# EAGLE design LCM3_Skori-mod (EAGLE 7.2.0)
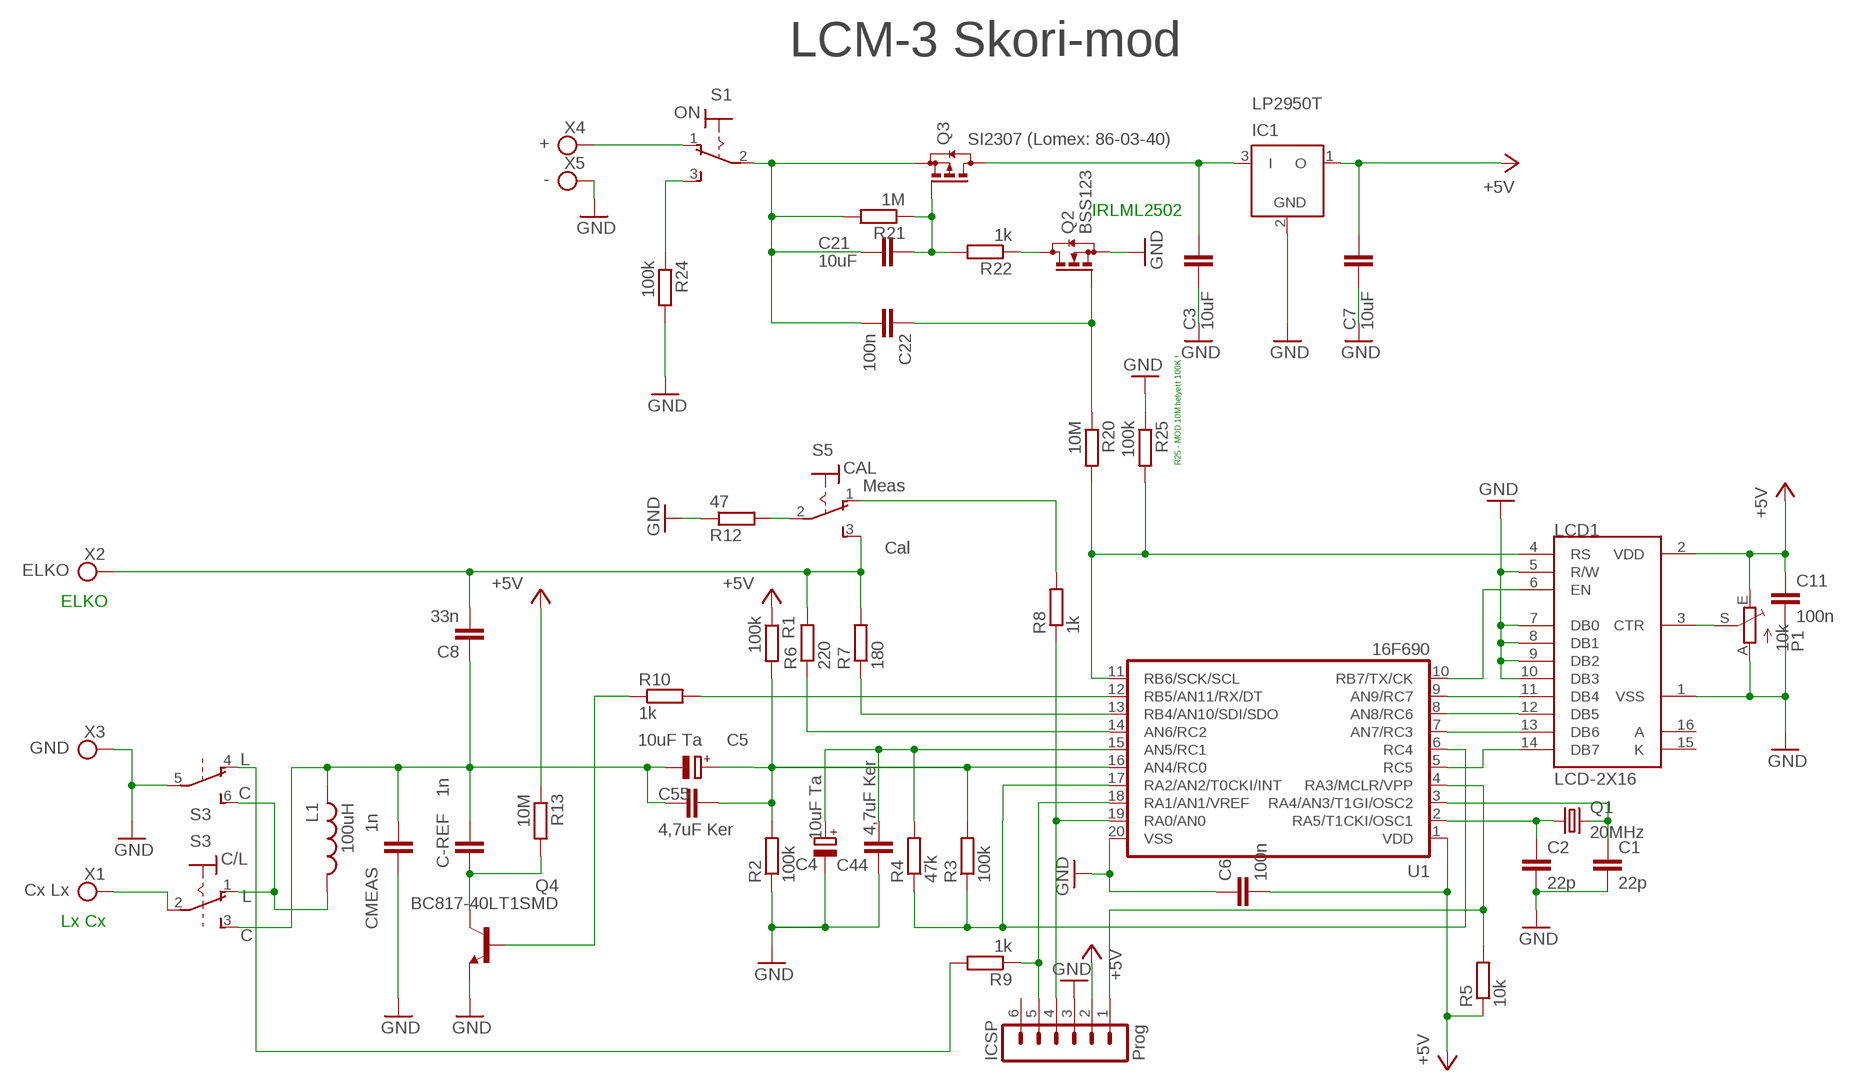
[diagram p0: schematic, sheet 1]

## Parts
C1  22p  C-EUC1206K  [C1206K]
C2  22p  C-EUC1206K  [C1206K]
C3  10uF  C-EUC1206K  [C1206K]
C4  10uF Ta  CPOL-EU085CS-1AR  [085CS_1AR]
C5  10uF Ta  CPOL-EU085CS-1AR  [085CS_1AR]
C6  100n  C-EUC1206K  [C1206K]
C7  10uF  C-EUC1206K  [C1206K]
C8  33n  C-EU102-064X133  [C102-064X133]
C11  100n  C-EUC1206K  [C1206K]
C21  10uF  C-EUC1206K  [C1206K]
C22  100n  C-EUC1206K  [C1206K]
C44  4,7uF Ker  C-EUC1206K  [C1206K]
C55  4,7uF Ker  C-EUC1206K  [C1206K]
C-REF  1n  C-EU102-064X133  [C102-064X133]
CMEAS  1n  C-EU102-064X133  [C102-064X133]
IC1  LP2950T  [TO92-T]
ICSP  Prog  MA06-1  [MA06-1]
L1  100uH  L-USTJ3-U2  [TJ3-U2]
LCD1  LCD-2X16  LCD-2X16,  [MTB-086]
P1  10k  TRIM_EU-CA9V  [CA9V]
Q1  20MHz  CRYSTALHC49U70  [HC49U70]
Q2  BSS123  [SOT23]
Q3  SI2307 (Lomex: 86-03-40)  BSS84  [SOT23]
Q4  BC817-40LT1SMD  [SOT23-BEC]
R1  100k  R-EU_R1206  [R1206]
R2  100k  R-EU_R1206  [R1206]
R3  100k  R-EU_R1206  [R1206]
R4  47k  R-EU_R1206  [R1206]
R5  10k  R-EU_R1206  [R1206]
R6  220  R-EU_R1206  [R1206]
R7  180  R-EU_R1206  [R1206]
R8  1k  R-EU_R1206  [R1206]
R9  1k  R-EU_R1206  [R1206]
R10  1k  R-EU_R1206  [R1206]
R12  47  R-EU_R2512  [R2512]
R13  10M  R-EU_R1206  [R1206]
R20  10M  R-EU_R1206  [R1206]
R21  1M  R-EU_R1206  [R1206]
R22  1k  R-EU_R1206  [R1206]
R24  100k  R-EU_R1206  [R1206]
R25  100k  R-EU_R1206  [R1206]
S1  ON  M9040P  [M9040P]
S3  C/L  M9040P2,  [M9040P2B]
S5  CAL  M9040P  [M9040P]
U1  16F690  PIC16F6XX  [DIL20]
X1  Cx Lx  PIN1,3-121  [PIN-4]
X2  ELKO  PIN1,3-121  [PIN-4]
X3  GND  PIN1,3-121  [PIN-4]
X4  +  PIN1,3-121  [PIN-4]
X5  -  PIN1,3-121  [PIN-4]

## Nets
+5V: C6.2 C7.1 C11.1 IC1.1(O) ICSP.2 LCD1.2(VDD) P1.E R1.1 R5.1 R13.1 U1.1(VDD)
GND: C1.2 C2.2 C3.2 C4.- C6.1 C7.2 C11.2 C44.1 CMEAS.1 IC1.2(GND) ICSP.3 LCD1.1(VSS) LCD1.5(R/W) LCD1.7(DB0) LCD1.8(DB1) LCD1.9(DB2) LCD1.10(DB3) P1.A Q2.2(S) Q4.E R2.1 R12.1 R24.2 R25.1 S3.5(2:P) U1.20(VSS) X3.1(KL) X5.1(KL)
N$1: LCD1.14(DB7) U1.5(RC5)
N$2: LCD1.13(DB6) U1.7(AN7/RC3)
N$3: LCD1.12(DB5) U1.8(AN8/RC6)
N$4: LCD1.11(DB4) U1.9(AN9/RC7)
N$5: LCD1.3(CTR) P1.S
N$6: LCD1.4(RS) R20.2 R25.2 U1.11(RB6/SCK/SCL)
N$7: LCD1.6(EN) U1.10(RB7/TX/CK)
N$8: C1.1 Q1.2 U1.3(RA4/AN3/T1GI/OSC2)
N$9: C2.1 Q1.1 U1.2(RA5/T1CKI/OSC1)
N$10: R24.1 S1.3(S)
N$11: R3.1 R4.1 U1.6(RC4) U1.17(RA2/AN2/T0CKI/INT)
N$12: C4.+ C44.2 R4.2 U1.15(AN5/RC1)
N$13: C5.- C8.1 C55.2 C-REF.2 CMEAS.2 L1.2 S3.3(1:S)
N$14: C8.2 R6.2 R7.2 S5.3(S) X2.1(KL)
N$15: R10.2 U1.12(RB5/AN11/RX/DT)
N$16: R6.1 U1.14(AN6/RC2)
N$17: C-REF.1 Q4.C R13.2
N$18: R7.1 U1.13(RB4/AN10/SDI/SDO)
N$19: ICSP.4 R8.1 U1.19(RA0/AN0)
N$20: R8.2 S5.1(O)
N$21: R12.2 S5.2(P)
N$22: ICSP.5 R9.1 U1.18(RA1/AN1/VREF)
N$23: R9.2 S3.4(2:O)
N$24: L1.1 S3.1(1:O) S3.6(2:S)
N$25: C5.+ C55.1 R1.2 R2.2 R3.2 U1.16(AN4/RC0)
N$26: S3.2(1:P) X1.1(KL)
N$27: ICSP.1 R5.2 U1.4(RA3/MCLR/VPP)
N$28: S1.1(O) X4.1(KL)
N$29: C3.1 IC1.3(I) Q3.3(D)
N$30: Q2.3(D) R22.1
N$31: C21.1 Q3.1(G) R21.1 R22.2
N$32: C21.2 C22.2 Q3.2(S) R21.2 S1.2(P)
N$34: C22.1 Q2.1(G) R20.1
N$37: Q4.B R10.1
Unconnected: ICSP.6

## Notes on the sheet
- LCM-3 Skori-mod
- IRLML2502
- R25 - MOD 10M helyett 100K !
- Meas
- Cal
- ELKO
- L
- C
- L
- Lx Cx
- C

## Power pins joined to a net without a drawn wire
A: LCD1.16(A)
K: LCD1.15(K)

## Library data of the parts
C1-C3 C6-C8 C11 C21 C22 C44 C55 C-REF CMEAS = rcl:C-EU: CAPACITOR, European symbol
C4 C5 = rcl:CPOL-EU: POLARIZED CAPACITOR, European symbol
IC1 = linear:LP2950: 100 mA, Low Power Low Dropout Voltage Regulator Source: http://www.onsemi.com/pub/Collateral/LP2950-D.PDF
ICSP = con-lstb:MA06-1: PIN HEADER
L1 = rcl:L-US: INDUCTOR, American symbol
LCD1 = 01_LCM3:LCD-2X16: LCD kijelzö
P1 = pot:TRIM_EU-: POTENTIOMETER
Q1 = crystal:CRYSTAL: CRYSTAL
Q2 = transistor-small-signal:BSS123: N-CHANNEL MOS FET
Q3 = transistor-small-signal:BSS84: P-CHANNEL MOS FET
Q4 = transistor-npn:BC817*: NPN Transistor
R1-R10 R12 R13 R20-R22 R24 R25 = rcl:R-EU_: RESISTOR, European symbol
S1 S5 = switch:M9040P: TOGGLE SWITCH Marquardt
S3 = 01_LCM3:M9040P2: TOGGLE SWITCH Marquardt
U1 = pic16f690:PIC16F6XX
X1-X5 = 01skori-hp:PIN: CONNECTOR

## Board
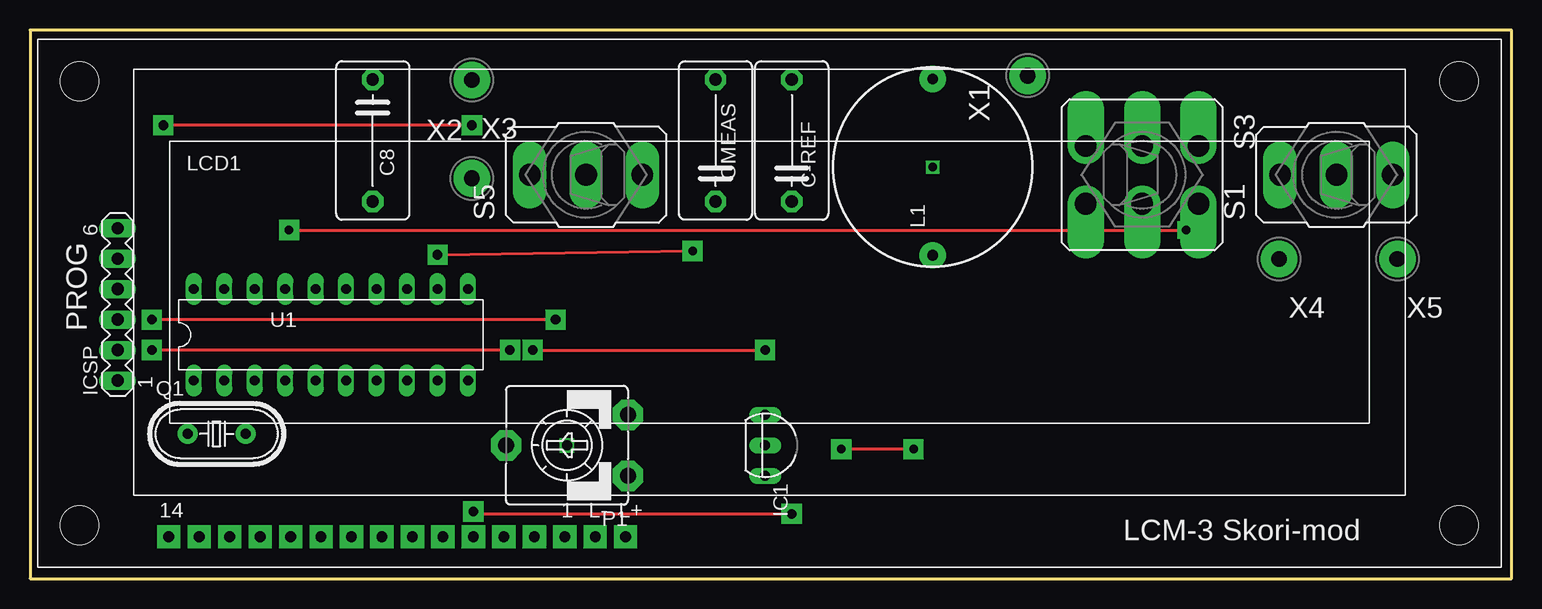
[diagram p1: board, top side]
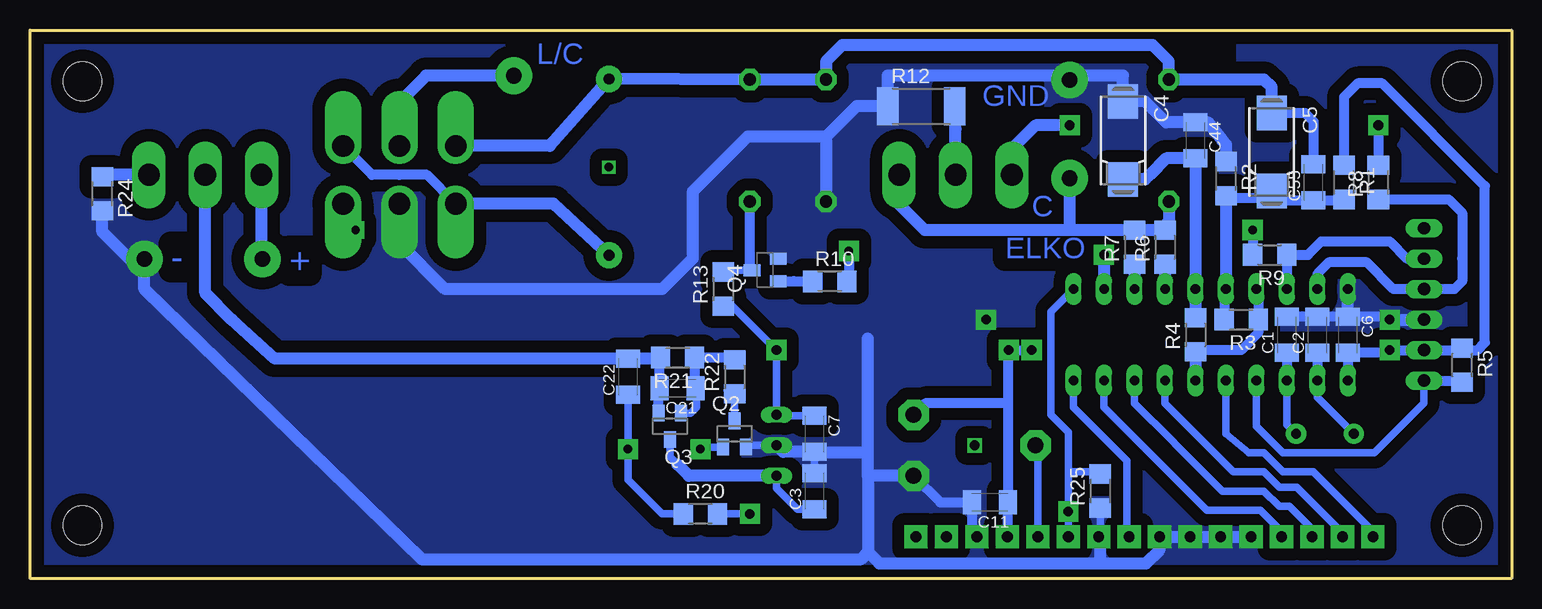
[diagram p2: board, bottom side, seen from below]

Size 123.51 x 45.72 mm. Coordinates in mm from the lower left corner, seen from the top.
Outline: 0,0 123.51,0 123.51,45.72 0,45.72 0,0
Copper layers (1*16): Top 0.035mm / dielectric 1.5mm / Bottom 0.035mm
Design rules "default": minimum track width 10mil, minimum drill 24mil, track to track 8mil, track to pad 8mil, pad to pad 8mil, via to via 8mil, smd to smd 8mil, copper to edge 40mil, drill to drill 8mil, minimum pad ring 10mil, minimum via ring 8mil, stop-mask expansion 4mil, vias tented up to drill 0mil, thermal gap 10mil

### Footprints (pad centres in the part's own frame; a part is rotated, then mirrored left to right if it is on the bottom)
C1206K = smd 1.5 x 2: 1 -1.5,0; 2 1.5,0
085CS_1AR = smd 2.9 x 2.5: + 3.25,0; - -3.25,0
C102-064X133 = drill 1.016 pad 1.778 octagon: 1 -5.08,0; 2 5.08,0
TO92-T = drill 0.813 long: 1 -2.54,0; 2 0,0; 3 2.54,0
MA06-1 = drill 1.016 long: 1 -6.35,0; 2 -3.81,0; 3 -1.27,0; 4 1.27,0; 5 3.81,0; 6 6.35,0
TJ3-U2 = drill 0.9 pad 2.184: 1 -7.35,0; 2 7.35,0
MTB-086 = drill 0.9 pad 1.93 square: 1 43.942,2.54; 2 41.402,2.54; 3 38.862,2.54; 4 36.322,2.54; 5 33.782,2.54; 6 31.242,2.54; 7 28.702,2.54; 8 26.162,2.54; 9 23.622,2.54; 10 21.082,2.54; 11 18.542,2.54; 12 16.002,2.54; 13 13.462,2.54; 14 10.922,2.54; 15 46.482,2.54; 16 49.022,2.54 | hole 3.2: 3.5,3.5; 3.5,40.5; 118.5,40.5; 118.5,3.5
CA9V = drill 1.321 pad 2.54 octagon: A -2.54,-5.08; E 2.54,-5.08; S 0,5.08
HC49U70 = drill 0.813 pad 1.676: 1 -2.413,0; 2 2.413,0
SOT23 = smd 1 x 1.4: 1 -0.95,-1.1; 2 0.95,-1.1; 3 0,1.1
SOT23-BEC = smd 1 x 1.4: B -0.95,-1.1; C 0,1.1; E 0.95,-1.1
R1206 = smd 1.6 x 1.803: 1 -1.422,0; 2 1.422,0
R2512 = smd 1.8 x 3.2: 1 -2.8,0; 2 2.8,0
M9040P = drill 1.803 pad 2.794 long: 1 0,4.699; 2 0,0; 3 0,-4.699
M9040P2B = drill 1.803 pad 3.048 offset: 1 -2.413,4.699; 2 -2.413,0; 3 -2.413,-4.699; 4 2.413,4.699; 5 2.413,0; 6 2.413,-4.699
DIL20 = drill 0.813 long: 1 -11.43,-3.81; 2 -8.89,-3.81; 3 -6.35,-3.81; 4 -3.81,-3.81; 5 -1.27,-3.81; 6 1.27,-3.81; 7 3.81,-3.81; 8 6.35,-3.81; 9 8.89,-3.81; 10 11.43,-3.81; 11 11.43,3.81; 12 8.89,3.81; 13 6.35,3.81; 14 3.81,3.81; 15 1.27,3.81; 16 -1.27,3.81; 17 -3.81,3.81; 18 -6.35,3.81; 19 -8.89,3.81; 20 -11.43,3.81
PIN-4 = drill 1.3 pad 3.048: 1 0,0.025

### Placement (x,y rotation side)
C1  18.73,20.32 90 bottom
C2  16.19,20.32 90 bottom
C3  58.1,7.3 90 bottom
C4  32.39,36.51 270 bottom
C5  20,35.56 270 bottom
C6  13.65,20.32 270 bottom
C7  58.1,12.06 270 bottom
C8  28.58,36.51 270 top
C11  43.5,6.35 180 bottom
C21  69.53,15.88 180 bottom
C22  73.66,16.83 90 bottom
C44  26.35,36.51 270 bottom
C55  16.51,33.02 90 bottom
C-REF  63.5,36.51 90 top
CMEAS  57.15,36.51 90 top
IC1  61.28,11.11 270 top
ICSP  7.3,22.86 90 top
L1  75.25,34.29 90 top
LCD1  0.64,0.95 0 top
P1  44.77,11.11 90 top
Q1  15.56,12.06 0 top
Q2  64.77,12.06 0 bottom
Q3  70.17,12.7 180 bottom
Q4  62.23,25.72 90 bottom
R1  13.97,33.02 270 bottom
R2  23.81,33.34 270 bottom
R3  22.54,21.59 180 bottom
R4  26.35,20.32 90 bottom
R5  4.13,17.78 270 bottom
R6  28.89,27.62 90 bottom
R7  31.43,27.62 90 bottom
R8  11.11,33.02 90 bottom
R9  20.16,26.99 180 bottom
R10  56.83,24.77 0 bottom
R12  49.21,39.37 0 bottom
R13  65.72,24.13 90 bottom
R20  67.63,5.4 0 bottom
R21  69.53,18.41 180 bottom
R22  64.77,16.83 90 bottom
R24  117.47,32.07 270 bottom
R25  34.29,7.3 90 bottom
S1  108.9,33.65 90 top
S3  92.71,33.65 270 top
S5  46.36,33.65 90 top
U1  25.08,20.32 0 top
X1  83.19,41.91 90 top
X2  36.83,33.34 0 top
X3  36.83,41.59 180 top
X4  104.14,26.67 180 top
X5  113.98,26.67 180 top

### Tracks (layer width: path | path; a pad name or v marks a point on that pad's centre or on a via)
+5V  (via drill 0.8 pad 1.68)
  Top 0.254: v40,19.05 v10.16,19.05 | v41.91,19.05 v61.28,19.05
  Bottom 0.61: C11.1 42.04,6.39 42.04,6.98 | C7.1 61.19,13.56 IC1.1 v61.28,19.05 64.94,22.71 R13.1
  Bottom 0.813: R1.1 13.97,40.13 12.83,41.27 10.8,41.27 2.22,32.7 2.22,19.68 2.86,19.05 3.66,19.05 R5.1 3.81,19.05 ICSP.2 v10.16,19.05 10.16,18.82 C6.2 U1.1 | 42,14.6 42,19.05 v41.91,19.05 v40,19.05 | 42,14.6 C11.1 | P1.E 48.9,14.6 42,14.6 | 42.04,6.98 LCD1.2
GND  (via drill 0.8 pad 1.68)
  Top 0.254: v43.81,21.59 v10.16,21.59
  Bottom 0.61: C11.2 44.58,5.93 | C7.2 58.1,10.48 C3.2 | R25.1 34.29,3.49 LCD1.5 | 73.34,1.59 73.49,1.59 | Q2.2 63.67,11.11 IC1.2
  Bottom 0.813: C4.- 32.46,39.76 | C1.2 C2.2 C6.1 10.16,21.82 v10.16,21.59 | 34.29,3.37 LCD1.5 | P1.A 47.62,6.35 C11.2 45,3.49 LCD1.1
  Bottom 1.016: LCD1.10 LCD1.9 LCD1.8 LCD1.7 29.34,2.41 30.48,1.27 34.29,1.27 | C6.1 U1.20 | v10.16,21.59 ICSP.3 | 23.81,34.61 R2.1 23.81,36.2 24.13,36.51 25.31,38.01 C44.1 28.81,38.01 30.56,39.76 C4.- 32.39,41.91 36.17,41.91 | 36.17,41.91 X3.1 | 36.17,41.91 52.01,41.91 R12.1 54.61,39.37 57.15,36.83 | 57.15,36.83 CMEAS.1 | 34.29,1.27 52.7,1.27 53.66,2.22 | 53.66,10.48 53.66,20 | 53.66,8.57 53.66,10.48 | 53.66,8.57 53.66,2.22 | P1.A 53.66,8.57 | 34.29,1.27 34.29,3.37 | 53.66,2.22 54.29,1.59 73.34,1.59 90.81,1.59 113.98,24.13 X5.1 114.01,26.67 115.25,26.67 117.47,28.89 R24.2 | IC1.2 60.73,10.56 C7.2 | 53.66,10.48 58.1,10.48 | S3.5 92.71,27.94 88.9,24.13 70.8,24.13 68.26,26.67 68.26,32.25 63.68,36.83 57.15,36.83
  pour Bottom (isolate 1.016, no thermals): 0.95,44.45 122.24,44.45 122.24,0.63 0.95,0.63
N$1
  Bottom 0.61: LCD1.14 11.75,3.68 11.75,4.13 16.51,8.89 19.05,8.89 20.64,10.48 21.91,10.48 23.81,12.06 23.81,13.65 U1.5
N$2
  Bottom 0.61: LCD1.13 14.29,3.68 14.29,4 17.91,7.62 19.05,7.62 19.37,7.62 20.64,8.89 23.18,8.89 26.35,12.06 27.31,13.02 28.89,14.6 28.89,15.24 U1.7
N$3
  Bottom 0.61: LCD1.12 16.83,3.68 16.83,4.32 18.54,6.03 18.73,6.03 19.37,6.03 20.64,7.3 21.91,7.3 24.13,7.3 27.94,11.11 28.26,11.43 31.43,14.6 U1.8
N$4
  Bottom 0.61: U1.9 33.97,14.29 29.53,9.84 25.4,5.72 20.95,5.72 19.69,4.45 19.18,3.94 LCD1.11
N$5
  Bottom 0.61: P1.S 39.5,10.92 LCD1.3
N$6  (via drill 0.8 pad 1.68)
  Top 0.254: 37.15,5.4 v63.5,5.4
  Top 0.61: v36.96,5.59 37.15,5.4
  Bottom 0.61: U1.11 38.42,22.23 38.42,21.59 38.42,13.65 36.96,12.19 36.96,8.89 | 36.96,8.89 v36.96,5.59 LCD1.4 | R25.2 34.29,8.89 36.96,8.89 | v63.5,5.4 R20.2
N$7
  Bottom 0.61: LCD1.6 32.07,3.68 32.07,9.84 36.51,14.29 U1.10
N$8
  Bottom 0.61: Q1.2 18.73,12.83 U1.3
  Bottom 0.813: C1.1 U1.3
N$9
  Bottom 0.61: Q1.1 16.19,15.11 U1.2
  Bottom 0.813: C2.1 U1.2
N$10
  Bottom 1.016: R24.1 117.31,33.65 S1.3
N$11
  Bottom 0.813: U1.17 21.12,23.98 R3.1 21.12,20.47 22.54,19.05 23.02,19.05 26.2,19.05 R4.1
  Bottom 1.016: R4.1 26.35,17.78 U1.6
N$12
  Bottom 1.016: R4.2 26.35,22.23 U1.15 C44.2 28.81,35.01 30.16,33.65 30.56,33.26 C4.+
N$13
  Bottom 0.813: 57.15,41.91 CMEAS.2 | C5.- 17.22,38.81 16.51,38.1 C55.2
  Bottom 1.016: CMEAS.2 C-REF.2 L1.2 80.18,36.07 S3.3 | 57.15,41.91 57.15,43.1 55.8,44.45 29.92,44.45 28.58,43.1 C8.1 20.64,41.59 20,40.96 C5.-
N$14
  Bottom 0.813: R6.2 28.89,29.53 28.58,29.85
  Bottom 1.016: R6.2 R7.2 33.17,29.04 36.83,29.04 | C8.2 28.58,29.85 | X2.1 36.83,30.48 36.83,29.04 | S5.3 51.05,31.19 48.91,29.04 36.83,29.04
N$15  (via drill 0.7 pad 1.68, 0.8 pad 1.68)
  Top 0.254: v33.97,26.99 v55.24,27.3
  Bottom 0.813: v55.24,27.3 55.24,24.93 R10.2
  Bottom 1.016: v33.97,26.99 U1.12
N$16
  Bottom 1.016: R6.1 U1.14
N$17
  Bottom 0.61: 63.5,25.72 65.56,25.72 arc-90 R13.2
  Bottom 0.813: Q4.C 63.5,25.72 C-REF.1
N$18
  Bottom 1.016: R7.1 U1.13
N$19
  Bottom 0.813: U1.19 16.19,25.4 15.24,26.35 12.06,26.35 9.84,24.13 ICSP.4 4.76,24.13 4.13,24.77 4.13,26.67 4.13,30.48 5.25,31.6 R8.1
N$20  (via drill 0.8 pad 1.68)
  Top 0.254: v36.83,37.78 v11.11,37.78
  Bottom 0.813: v11.11,37.78 R8.2
  Bottom 1.016: v36.83,37.78 39.69,37.78 41.59,35.88 S5.1
N$21
  Bottom 1.016: R12.2 46.36,37.46 S5.2
N$22
  Bottom 0.813: U1.18 R9.1 16.99,26.99 15.88,28.1 14.76,28.1 10.16,28.1 8.73,26.67 ICSP.5
N$23  (via drill 0.7 pad 1.42, 0.7 pad 1.68)
  Top 0.254: v21.59,29.05 v96.36,29.05
  Bottom 0.813: R9.2 21.59,28.58 v21.59,29.05
  Bottom 1.016: S3.4 96.36,29.02 v96.36,29.05
N$24
  Bottom 0.813: S3.1 95,33.65 92.71,33.65 90.42,33.65 S3.6
  Bottom 1.016: S3.6 87.76,31.24 79.87,31.24 L1.1
N$25
  Bottom 0.813: R1.2 13.73,31.52 C55.1 20,31.52 20,31.75 | 20,31.75 C5.+ | R2.2 23.5,31.75 20,31.75 | U1.16 23.97,23.98 R3.2
  Bottom 1.016: R2.2 U1.16
N$26
  Bottom 1.016: X1.1 83.16,41.88 83.19,41.91 89.85,41.91 90.49,41.91 92.71,39.69 S3.2
N$27
  Bottom 0.61: U1.4 21.27,13.97 21.27,12.7 19.05,10.48 11.43,10.48 7.3,14.6 ICSP.1
  Bottom 0.813: R5.2 arc-90 3.96,16.51 ICSP.1
N$28
  Bottom 1.016: X4.1 104.2,26.71 S1.1
N$29
  Bottom 0.61: C3.1 59.54,5.8 61.28,7.54 IC1.3 | 69.53,9.52 70.17,10.16 Q3.3
  Bottom 1.016: IC1.3 68.58,8.57 69.53,9.52
N$30
  Bottom 0.61: R22.1 65.41,15.71 64.77,15.56 64.77,15.24 Q2.3
N$31
  Bottom 0.61: Q3.1 68.43,13.8 67.94,14.29 67.94,15.88 C21.1 | R22.2 64.77,18.41
  Bottom 0.813: C21.1 68.11,15.88 R21.1 64.77,18.41 R22.2
N$32
  Bottom 0.61: 71.12,15.88 C21.2
  Bottom 0.813: 71.12,15.88 Q3.2 | C21.2 71.03,18.41
  Bottom 1.016: 71.03,18.41 R21.2 71.04,18.33 C22.2 79.06,18.33 103.1,18.33 106.68,21.59 108.9,23.81 S1.2
N$33  (via drill 0.7)
  other vias: 75.25,34.29
N$34  (via drill 0.7 pad 1.68)
  Top 0.254: v73.66,10.8 v67.63,10.8
  Bottom 0.61: R20.1 70.8,5.4 73.66,8.26 C22.1 v73.66,10.8 | v67.63,10.8 67.48,10.94 Q2.1
N$35  (via drill 0.8)
  other vias: 44.77,11.11
N$36
  pour Bottom (isolate 1.016): 1.27,44.77 22.86,44.77 22.86,31.43 0.64,31.43 0.64,44.77
N$37
  Bottom 0.813: Q4.B 59.86,24.78 R10.1

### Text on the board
Bottom: L/C | GND | C | ELKO | + | -
tPlace: PROG | LCM-3 Skori-mod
